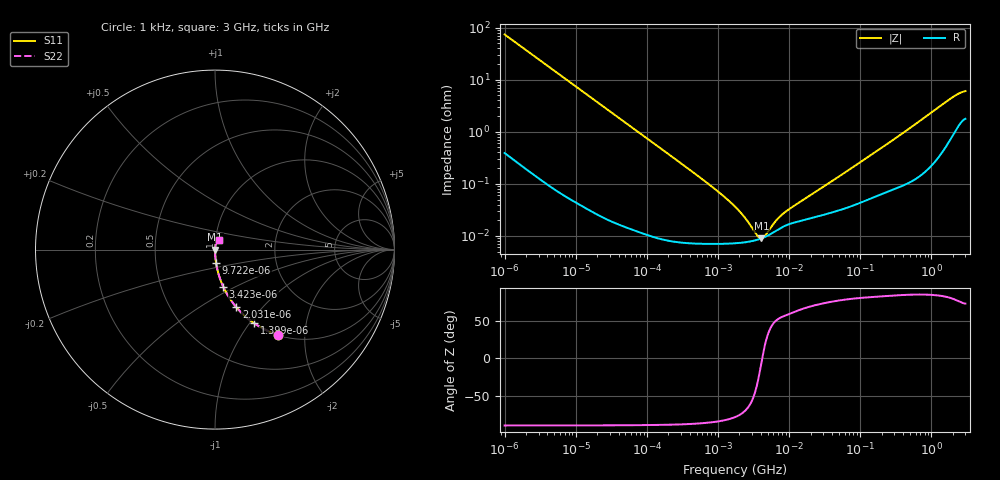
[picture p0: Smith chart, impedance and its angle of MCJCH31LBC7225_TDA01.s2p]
! MCJCH31LBC7225_TDA01  S-PARAMETER MODEL  ( Standard Model )
! Model Generated by TAIYO YUDEN Corporation (http://www.ty-top.com)
! Version 1.0
! TAIYO YUDEN Control No. 220601
! Copyright(c) 2016 TAIYO YUDEN CO.,LTD. All Rights Reserved.
! Product Description (link to TY-COMPAS)
! https://ds.yuden.co.jp/TYCOMPAS/or/detail?pn=MCJCH31LBC7225KTDA01&u=M
! Products Name : Multilayer Ceramic Capacitors
! Characteristics :
!  Capacitance : 2.2 [uF] , Rated Voltage : 100 [V] , TCC : X7S
!  Case Size : 3.2 x 1.6 / 0.126 x 0.063 [mm/inch] , Thickness : 1.6 / 0.063 [mm/inch]
!  (Conditions: Temperature = 25 [degC] , DC Bias Voltage = 0 [V])
! External Node Assignments :
!  1  o---| |---o  2
! GND o---------o GND
! Frequency Range : 1kHz  -  3GHz  [ 401 STEP ]
# MHZ S RI R 50
! Freq[MHz].  S11 Real  S11 Imag  S21 Real  S21 Imag  S12 Real  S12 Imag  S22 Real  S22 Imag
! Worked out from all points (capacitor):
!   401 points, 1 kHz to 3 GHz, reference 50 ohm
!   read as one part in series: C = 2.16 uF near 1.077 kHz
!   lowest |Z| = 9.02 mohm at 4.083 MHz (marker M1)
!   series resonance near 4.185 MHz, so ESL is about 670 pH
!   S11 on the Smith chart (normalised r, x): 1 kHz: 1.01, -1.47; 1.399 kHz: 1.01, -1.06; 2.031 kHz: 1.00, -0.73; 3.423 kHz: 1.00, -0.43; 9.722 kHz: 1.00, -0.15; 3 GHz: 1.04, +0.12
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0.001  0.3527 -0.4752  0.6473 0.4752  0.6473 0.4752  0.3527 -0.4752
0.001399  0.2189 -0.4109  0.7811 0.4109  0.7811 0.4109  0.2189 -0.4109
0.002031  0.1181 -0.3202  0.8819 0.3202  0.8819 0.3202  0.1181 -0.3202
0.003423  0.0456 -0.2061  0.9544 0.2061  0.9544 0.2061  0.0456 -0.2061
0.009722  0.00623 -0.0758  0.9938 0.0758  0.9938 0.0758  0.00623 -0.0758
0.01216  0.00409 -0.0608  0.9959 0.0608  0.9959 0.0608  0.00409 -0.0608
0.033275  0.000685 -0.0224  0.9993 0.0224  0.9993 0.0224  0.000685 -0.0224
0.147855  0.000114 -0.00506  0.9999 0.00506  0.9999 0.00506  0.000114 -0.00506
0.791611  7.1e-05 -0.000914  0.9999 0.000914  0.9999 0.000914  7.1e-05 -0.000914
1.732051  7.24e-05 -0.000358  0.9999 0.000358  0.9999 0.000358  7.24e-05 -0.000358
2.422679  7.56e-05 -0.000205  0.9999 0.000205  0.9999 0.000205  7.56e-05 -0.000205
3.388684  8.27e-05 -7.53e-05  0.9999 7.53e-05  0.9999 7.53e-05  8.27e-05 -7.53e-05
3.651041  8.52e-05 -4.83e-05  0.9999 4.83e-05  0.9999 4.83e-05  8.52e-05 -4.83e-05
4.083148  8.97e-05 -8.59e-06  0.9999 8.59e-06  0.9999 8.59e-06  8.97e-05 -8.59e-06
4.739869  9.79e-05 4.33e-05  0.9999 -4.33e-05  0.9999 -4.33e-05  9.79e-05 4.33e-05
6.387174  0.000123 0.000143  0.9999 -0.000143  0.9999 -0.000143  0.000123 0.000143
8.291982  0.000151 0.000224  0.9998 -0.000224  0.9998 -0.000224  0.000151 0.000224
21.06097  0.000222 0.0006  0.9998 -0.0006  0.9998 -0.0006  0.000222 0.0006
256.0921  0.000764 0.00617  0.9992 -0.00617  0.9992 -0.00617  0.000764 0.00617
1917.819  0.00958 0.0432  0.9904 -0.0432  0.9904 -0.0432  0.00958 0.0432
2489.759  0.0164 0.0519  0.9836 -0.0519  0.9836 -0.0519  0.0164 0.0519
3000  0.0206 0.0555  0.9794 -0.0555  0.9794 -0.0555  0.0206 0.0555
